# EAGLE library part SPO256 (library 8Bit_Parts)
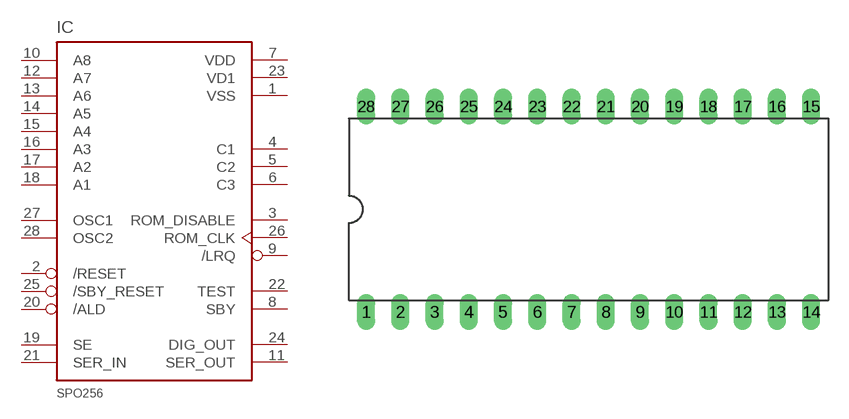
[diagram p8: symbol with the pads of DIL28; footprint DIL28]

Designator prefix IC

## SPO256  [DIL28]
1  VSS  pwr
2  /RESET  in
3  ROM_DISABLE  out
4  C1  out
5  C2  out
6  C3  out
7  VDD  pwr
8  SBY  out
9  /LRQ  out
10  A8  in
11  SER_OUT  out
12  A7  in
13  A6  in
14  A5  in
15  A4  in
16  A3  in
17  A2  in
18  A1  in
19  SE  in
20  /ALD  in
21  SER_IN  in
22  TEST  nc
23  VD1  pwr
24  DIG_OUT  out
25  /SBY_RESET  in
26  ROM_CLK  out
27  OSC1  in
28  OSC2  in

## Footprint DIL28 (pad centres in mm)
Dual In Line Package
drill 0.813 long: 1 -16.51,-7.62; 2 -13.97,-7.62; 3 -11.43,-7.62; 4 -8.89,-7.62; 5 -6.35,-7.62; 6 -3.81,-7.62; 7 -1.27,-7.62; 8 1.27,-7.62; 9 3.81,-7.62; 10 6.35,-7.62; 11 8.89,-7.62; 12 11.43,-7.62; 13 13.97,-7.62; 14 16.51,-7.62; 15 16.51,7.62; 16 13.97,7.62; 17 11.43,7.62; 18 8.89,7.62; 19 6.35,7.62; 20 3.81,7.62; 21 1.27,7.62; 22 -1.27,7.62; 23 -3.81,7.62; 24 -6.35,7.62; 25 -8.89,7.62; 26 -11.43,7.62; 27 -13.97,7.62; 28 -16.51,7.62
